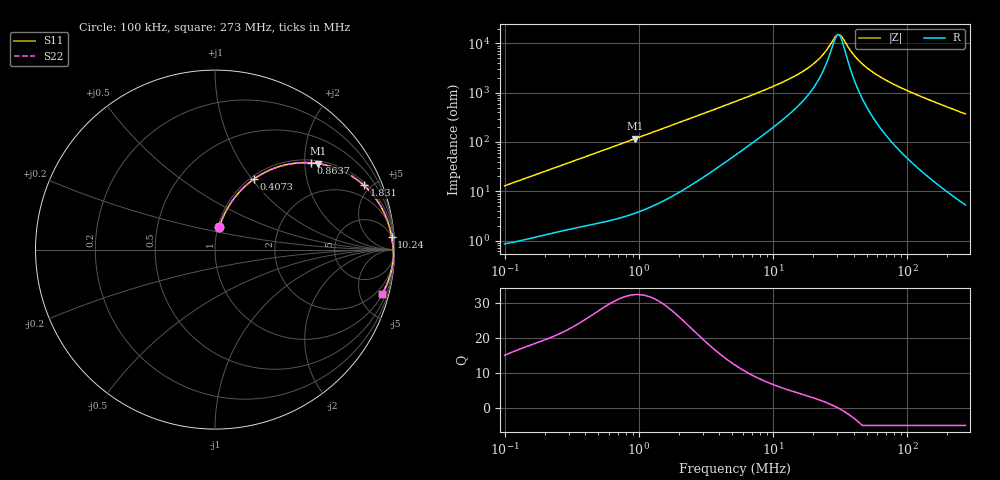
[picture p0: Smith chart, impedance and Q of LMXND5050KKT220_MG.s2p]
! LMXND5050KKT220_MG  S-PARAMETER MODEL  ( General Type )
! Model Generated by TAIYO YUDEN Corporation (http://www.ty-top.com)
! Version 1.0
! TAIYO YUDEN Control No. 191023NI43SB-FBB
! Copyright(c) 2019 TAIYO YUDEN CO.,LTD. All Rights Reserved.
! Product Description (link to TY-COMPAS)
! https://ds.yuden.co.jp/TYCOMPAS/or/detail?pn=LMXND5050KKT220MMG&u=M
! Products Name : Inductors
! Characteristics :
!  Inductance : 22 uH , SRF(min) : 15 MHz , DC Resistance(max) : 0.72 Ohm
!  Rated Current : Saturation :550 mA , Temp Rise : 450 mA
!  Case Size : 4.9 x 4.9 / 0.193 x 0.193 [mm/inch] , Thickness : 1 / 0.039 [mm/inch]
!  (Conditions: Temperature = 25 degC , DC Bias Current/Voltage = 0A / 0V)
! External Node Assignments :
!  1  o---GGG---o  2
! GND o---------o GND
! Frequency Range : 0.1MHz  -  272.98108MHz  [ 402 STEP ]
# MHz S RI R 50
! Freq[MHz].  S11 Real  S11 Imag  S21 Real  S21 Imag  S12 Real  S12 Imag  S22 Real  S22 Imag
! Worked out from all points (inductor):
!   401 points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, 100 kHz to 273 MHz, reference 50 ohm
!   read as one part in series: L = 20.4 uH near 104 kHz
!   highest Q = 32.5 at 934.8 kHz (marker M1), where L = 19.8 uH
!   self-resonance near 30.38 MHz
!   S11 on the Smith chart (normalised r, x): 100 kHz: 1.02, +0.26; 407.3 kHz: 1.04, +1.02; 863.7 kHz: 1.07, +2.15; 1.831 MHz: 1.17, +4.54; 10.24 MHz: 5, +27; 273 MHz: 1.11, -7.43
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0.1  0.0244 0.1248  0.9756 -0.1248  0.9756 -0.1248  0.0244 0.1248
0.212047  0.0785 0.245  0.9215 -0.245  0.9215 -0.245  0.0785 0.245
0.376316  0.192 0.3742  0.808 -0.3742  0.808 -0.3742  0.192 0.3742
0.407299  0.2157 0.3922  0.7843 -0.3922  0.7843 -0.3922  0.2157 0.3922
0.863667  0.5342 0.4836  0.4658 -0.4836  0.4658 -0.4836  0.5342 0.4836
0.934776  0.572 0.4796  0.428 -0.4796  0.428 -0.4796  0.572 0.4796
1.416134  0.7485 0.4179  0.2515 -0.4179  0.2515 -0.4179  0.7485 0.4179
1.831381  0.8291 0.3586  0.1709 -0.3586  0.1709 -0.3586  0.8291 0.3586
2.94406  0.9201 0.2473  0.0799 -0.2473  0.0799 -0.2473  0.9201 0.2473
5.329134  0.9672 0.1416  0.0328 -0.1416  0.0328 -0.1416  0.9672 0.1416
10.23617  0.9842 0.0701  0.0158 -0.0701  0.0158 -0.0701  0.9842 0.0701
14.90575  0.9886 0.0424  0.0114 -0.0424  0.0114 -0.0424  0.9886 0.0424
19.66158  0.9909 0.0254  0.00912 -0.0254  0.00912 -0.0254  0.9909 0.0254
23.0325  0.992 0.0163  0.00804 -0.0163  0.00804 -0.0163  0.992 0.0163
29.20284  0.9933 0.00279  0.00675 -0.00279  0.00675 -0.00279  0.9933 0.00279
30.98818  0.9935 -0.000608  0.0065 0.000608  0.0065 0.000608  0.9935 -0.000608
32.88267  0.9937 -0.00404  0.00628 0.00404  0.00628 0.00404  0.9937 -0.00404
39.28982  0.9942 -0.0146  0.00582 0.0146  0.00582 0.0146  0.9942 -0.0146
46.02595  0.9943 -0.0246  0.00572 0.0246  0.00572 0.0246  0.9943 -0.0246
73.9896  0.9923 -0.0597  0.00773 0.0597  0.00773 0.0597  0.9923 -0.0597
131.3077  0.9815 -0.1208  0.0185 0.1208  0.0185 0.1208  0.9815 -0.1208
272.9811  0.9294 -0.2491  0.0706 0.2491  0.0706 0.2491  0.9294 -0.2491
